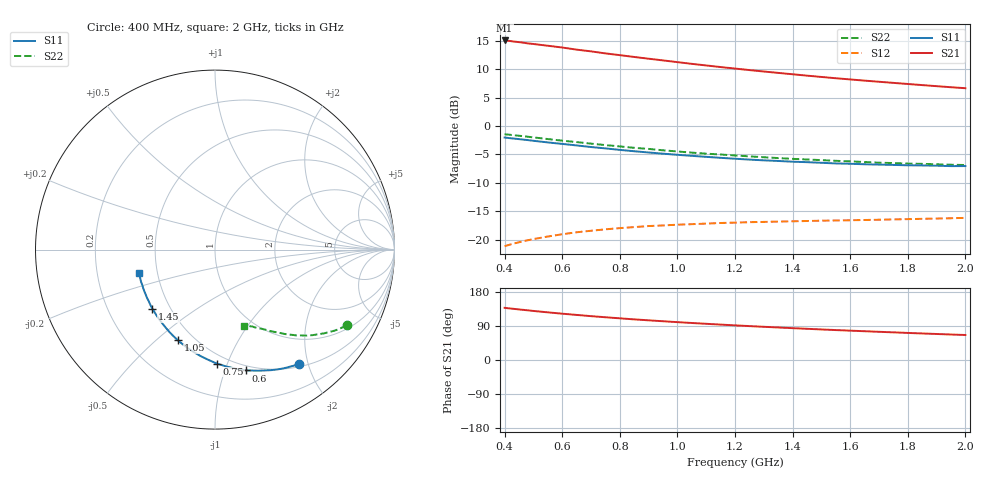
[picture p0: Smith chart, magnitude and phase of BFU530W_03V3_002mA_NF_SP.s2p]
! Filename:  P:\Prog\Test\Noise\ATS_data\Testdata_Net\06 Compressed Noise after Statistics\BFU530W_APM2013_09_A05_03p3V_002mA_NF_CM01_D.sf
! Date/Time: Tue 26/Mar/2013 18:06:08
! BFU530W_APM2013_09_A05_03p3V_1to25mA_NF_CM01_Bias2_R.sf
! Noise Parameter Data File
! BFU530W_APM2013_09_A05_03p3V_1to25mA_NF_CM01
! Date/time: Thu Mar 21 19:18:02 2013
! VAR V_out= 3.300000
! VAR I_out= 1.995000
! VAR V_in= 0.800300
! VAR I_in= 0.020905
! Device data file deembeded for feedlines and parallel
! Original file: \06 Compressed Noise after Statistics\BFU530W_APM2013_09_A05_03p3V_002mA_NF_CM01_R.sf
! Feed-files: PR019V01_070313_Feed1.s2p, PR019V01_070313_Feed2.s2p
! Parallel-file: PR019V01_070313_Par.s2p
# MHz S MA R 50
!  Freq-MHz  S11-mag  S11-arg  S21-mag  S21-arg  S12-mag  S12-arg  S22-mag  S22-arg
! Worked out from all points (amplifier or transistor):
!   37 points, 400 MHz to 2 GHz, reference 50 ohm
!   highest |S21| = 15.1 dB at 400 MHz (marker M1)
!   |S21| within 3 dB of that: start of sweep to 865.5 MHz
!   unconditionally stable (mu >= 1): nowhere
!   at 500 MHz: K = 0.28, MSG = 17.2 dB, |S12| = -19.9 dB
!   at 1.1 GHz: K = 0.58, MSG = 13.9 dB, |S12| = -17.2 dB
!   at 2 GHz: K = 0.94, MSG = 11.4 dB, |S12| = -16.2 dB
!   lowest NFmin = 0.49 dB at 420 MHz
!   S11 on the Smith chart (normalised r, x): 400 MHz: 0.54, -1.85; 600 MHz: 0.46, -1.19; 750 MHz: 0.43, -0.92; 1.05 GHz: 0.41, -0.59; 1.45 GHz: 0.40, -0.34; 2 GHz: 0.39, -0.13
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400  0.7912 -53.7  5.661 137.7  0.08747 59.7  0.8461 -29.9
420  0.7802 -56.1  5.594 135.9  0.09051 58.5  0.8357 -31.0
460  0.761 -60.7  5.431 132.7  0.09603 56.4  0.8153 -33.1
480  0.7513 -62.8  5.336 131.1  0.09856 55.4  0.8045 -34.1
500  0.7407 -65.1  5.271 129.5  0.101 54.5  0.7933 -35.1
550  0.7167 -70.3  5.085 125.8  0.1064 52.3  0.7672 -37.4
600  0.6952 -75.5  4.907 122.2  0.1114 50.3  0.7426 -39.5
650  0.674 -80.1  4.699 119.0  0.1159 48.5  0.7218 -41.3
700  0.6525 -84.8  4.538 115.7  0.1195 46.9  0.6991 -43.3
750  0.6349 -89.1  4.354 112.8  0.123 45.5  0.6789 -44.8
850  0.5991 -97.6  4.052 107.2  0.1288 43.1  0.6423 -47.7
950  0.5703 -105.1  3.778 102.3  0.1331 41.2  0.6106 -50.4
1050  0.5458 -112.3  3.523 97.7  0.1366 39.8  0.5827 -52.6
1150  0.5243 -119.1  3.301 93.4  0.1399 38.6  0.5608 -54.6
1200  0.5147 -122.1  3.203 91.4  0.1409 38.3  0.5498 -55.7
1300  0.4982 -128.3  3.017 87.6  0.143 37.8  0.5305 -57.5
1450  0.4801 -136.6  2.774 82.3  0.1457 37.5  0.5069 -60.1
1500  0.4741 -139.4  2.702 80.6  0.1466 37.4  0.5005 -61.1
1600  0.4646 -144.6  2.569 77.5  0.1479 37.7  0.4879 -62.7
1750  0.4542 -151.7  2.396 73.0  0.1505 38.5  0.4718 -65.0
1850  0.4494 -156.3  2.291 70.0  0.1523 39.0  0.4641 -66.6
2000  0.4436 -162.9  2.15 66.0  0.1552 40.3  0.4532 -69.1
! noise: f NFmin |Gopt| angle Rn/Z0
400  0.5279  0.4555  23.35  0.1826
460  0.5145  0.4593  29.87  0.1823
600  0.5585  0.4644  38.2  0.1832
800  0.5998  0.4636  53.45  0.1603
1000  0.6699  0.4709  64.09  0.161
1200  0.7061  0.4635  78.2  0.1448
1400  0.7328  0.4737  91.04  0.1206
1600  0.6592  0.4506  105.5  0.1041
1800  0.7839  0.4635  117.1  0.0963
2000  0.8644  0.4507  132.5  0.0796
